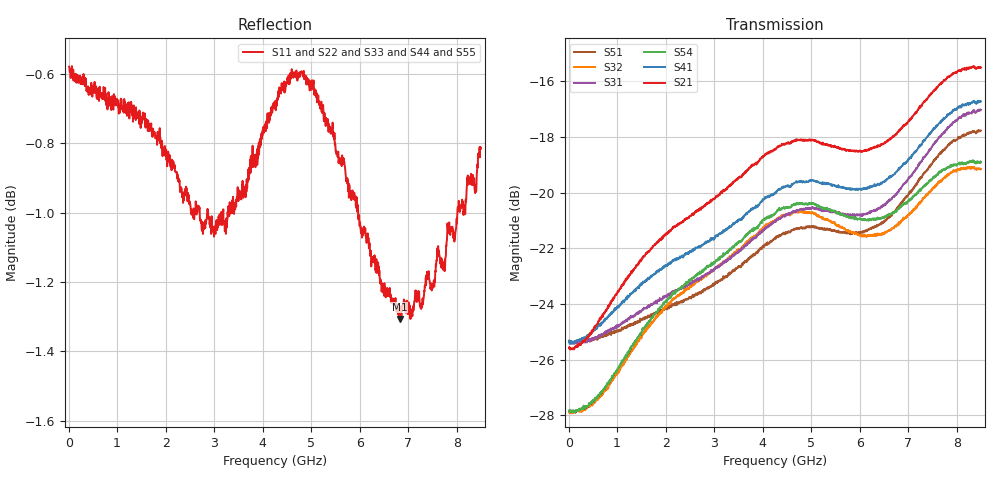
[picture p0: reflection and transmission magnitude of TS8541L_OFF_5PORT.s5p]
! Created with skrf (http://scikit-rf.org).
# Hz S RI R 50.0
!freq ReS11 ImS11 ReS12 ImS12 ReS13 ImS13
! ReS14 ImS14 ReS15 ImS15
! ReS21 ImS21 ReS22 ImS22 ReS23 ImS23
! ReS24 ImS24 ReS25 ImS25
! ReS31 ImS31 ReS32 ImS32 ReS33 ImS33
! ReS34 ImS34 ReS35 ImS35
! ReS41 ImS41 ReS42 ImS42 ReS43 ImS43
! ReS44 ImS44 ReS45 ImS45
! ReS51 ImS51 ReS52 ImS52 ReS53 ImS53
! ReS54 ImS54 ReS55 ImS55
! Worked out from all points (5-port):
!   1601 points, 10 MHz to 8.5 GHz, reference 50 ohm
!   strongest paths, dB at 10 MHz, 2.132 GHz, 4.255 GHz, 6.378 GHz, 8.5 GHz:
!     S21: -25.6, -21.3, -18.4, -18.3, -15.5
!     S41: -25.4, -22.5, -20.0, -19.7, -16.7
!     S54: -27.9, -23.6, -20.7, -20.9, -18.9
!     S31: -25.4, -23.6, -21.0, -20.6, -17.0
!     S32: -27.9, -23.9, -21.0, -21.5, -19.1
!     S51: -25.3, -24.0, -21.6, -21.2, -17.8
!   lowest |S11| = -1.3 dB at 6.823 GHz (marker M1), VSWR 13.32, Z = 9.67 + j62.3 ohm
!   |S11| at or under -10 dB: nowhere
